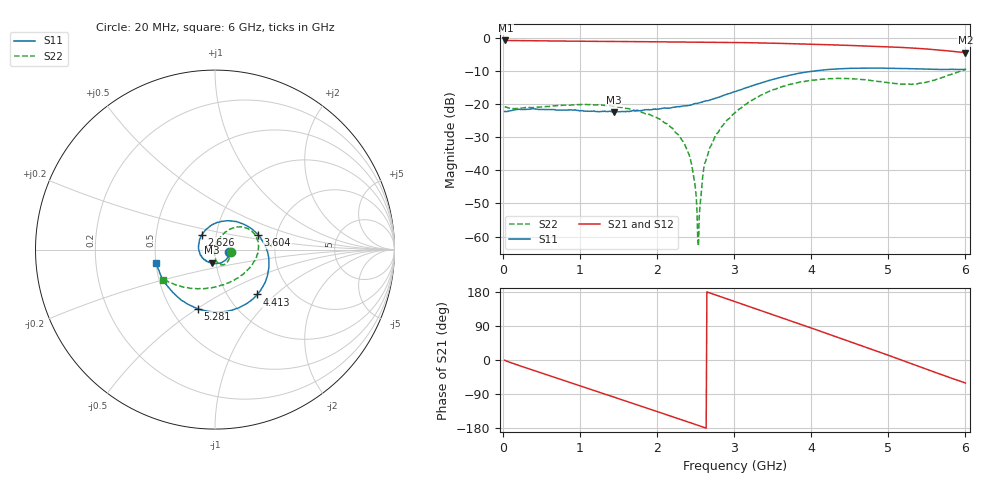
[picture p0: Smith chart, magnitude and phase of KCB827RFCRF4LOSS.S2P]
!Agilent Technologies,E5071B,JP1KK00126,A.08.11
!Date: Tue May 06 07:08:52 2014
!Data & Calibration Information:
!Freq	S11:SOLT2(ON)	S21:SOLT2(ON)	S12:SOLT2(ON)	S22:SOLT2(ON)
# Hz S dB R 50
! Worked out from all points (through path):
!   600 points, 20 MHz to 6 GHz, reference 50 ohm
!   highest |S21| = -0.78 dB at 29.98 MHz (marker M1); lowest = -4.4 dB at 6 GHz (marker M2)
!   group delay of S21, straight-line fit = 194 ps
!   lowest |S11| = -22.4 dB at 1.438 GHz (marker M3), VSWR 1.16, Z = 47.8 - j7.09 ohm
!   |S11| at or under -10 dB: start of sweep to 4.041 GHz
!   |S22| runs from -62.9 to -9.5 dB; largest |S21 - S12| = 0.0037
!   S11 on the Smith chart (normalised r, x): 20 MHz: 1.16, -0.04; 2.626 GHz: 0.85, +0.14; 3.604 GHz: 1.60, +0.28; 4.413 GHz: 1.36, -0.77; 5.281 GHz: 0.68, -0.50; 6 GHz: 0.50, -0.08
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2e7  -22.23 -11.6  -0.78 -0.5  -0.77 -0.6  -20.78 -9.1
2.998331e7  -22.25 -8.9  -0.78 -1.5  -0.77 -1.6  -20.87 -6.4
4.892154e8  -21.59 -35.4  -0.90 -33.7  -0.90 -33.7  -20.90 -25.6
1.018331e9  -21.97 -73.3  -1.00 -69.5  -1.01 -69.5  -20.10 -50.2
1.437629e9  -22.42 -103.1  -1.09 -97.7  -1.08 -97.9  -20.69 -67.4
2.016661e9  -21.53 -154.0  -1.19 -137.2  -1.18 -137.2  -24.39 -85.3
2.206344e9  -20.98 -175.1  -1.21 -150.2  -1.21 -150.2  -27.55 -90.0
2.386043e9  -20.49 163.0  -1.24 -162.6  -1.24 -162.5  -33.75 -95.6
2.46591e9  -20.05 151.9  -1.26 -168.1  -1.26 -168.1  -40.79 -100.0
2.505843e9  -19.77 146.5  -1.27 -170.7  -1.27 -170.8  -47.74 -87.4
2.535793e9  -19.69 142.8  -1.26 -172.8  -1.27 -173.0  -62.92 106.4
2.55576e9  -19.56 140.2  -1.27 -174.2  -1.27 -174.3  -50.78 102.3
2.58571e9  -19.39 136.0  -1.28 -176.4  -1.28 -176.3  -43.14 73.6
2.625643e9  -19.08 131.2  -1.29 -179.0  -1.29 -179.1  -37.51 77.9
2.775392e9  -18.10 111.5  -1.32 170.5  -1.32 170.4  -28.85 74.3
3.014992e9  -16.21 81.9  -1.39 153.8  -1.38 153.7  -22.51 66.3
3.604007e9  -11.92 18.9  -1.66 112.3  -1.66 112.2  -14.90 44.5
4.013322e9  -10.07 -16.3  -1.93 83.4  -1.94 83.4  -12.76 26.6
4.412654e9  -9.29 -46.7  -2.21 55.0  -2.22 55.0  -12.29 6.2
5.011653e9  -9.17 -87.1  -2.70 11.6  -2.70 11.6  -13.61 -38.3
5.281202e9  -9.31 -106.0  -3.02 -8.4  -3.03 -8.4  -13.99 -69.0
6e9  -9.48 -167.6  -4.44 -60.7  -4.45 -60.6  -9.54 -150.0
